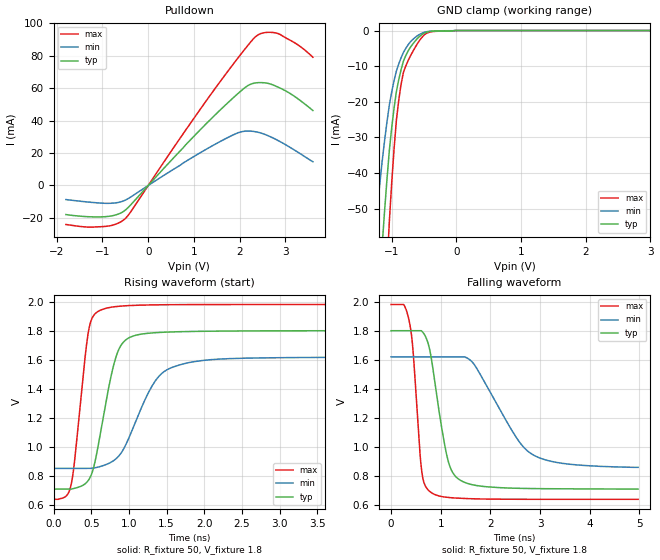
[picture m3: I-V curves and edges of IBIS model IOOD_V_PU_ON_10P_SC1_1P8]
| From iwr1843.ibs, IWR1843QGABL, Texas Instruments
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|   Model Cell IOOD_V_PU_ON_10P_SC1_1P8
|IOOD_V_PU_ON_10P_SC1_1P8
[Model]   IOOD_V_PU_ON_10P_SC1_1P8
Model_type   I/O_open_drain
Polarity   Non-Inverting
Enable   Active-Low
Vinl =  0.63
Vinh =  1.17
Cref =  15pF
Rref =  100.0000M
Vref =  0V
Vmeas =  0.9
|   typ   min   max
C_comp   2.290246p   2.205796p   2.292736p
[Model Spec]
Vinl   0.63   0.567   0.693
Vinh   1.17   1.053   1.287
[Temperature Range]   25   125   -40
[Voltage Range]   1.8   1.62   1.98
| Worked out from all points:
|   slope of the pulldown table from 0 to 0.27 V, typ, clamps not added: 32.2 ohm
|   GND clamp passes 1 mA (typ) near -0.52 V on its own axis
|   rising waveform, R_fixture 50, V_fixture 1.8: 20-80 % time 245ps typ, 416ps min, 160ps max; typ from 0.711 V to 1.8 V
|   falling waveform, R_fixture 50, V_fixture 1.8: 20-80 % time 308ps typ, 788ps min, 165ps max; typ from 1.8 V to 0.71 V
| Where Nom  PVT is Nominal Process, 1.8V, 25C
|   Fast PVT is Strong Process,  1.98V, -40C
|   Slow PVT is Weak Process,   1.62V, 125C
[Pulldown]
|   voltage   I(typ)   I(min)   I(max)
-1.8V     -17.92mA   -8.674mA   -24.03mA
-927.3mV  -19.22mA   -10.99mA   -25.21mA
-654.5mV  -17.65mA   -10.46mA   -23.22mA
-490.9mV  -14.97mA   -8.904mA   -20.12mA
818.2mV   25.06mA    14.78mA    34.16mA
1.691V    49.7mA     28.87mA    68.59mA
2.127V    60.63mA    33.53mA    84.59mA
2.4V      63.43mA    32.84mA    92.9mA
2.618V    62.99mA    30.74mA    94.47mA
2.836V    60.69mA    27.76mA    93.76mA
3.273V    53.49mA    20.53mA    86.73mA
3.6V      46.26mA    14.64mA    79.12mA
[GND_clamp]
|   voltage   I(typ)   I(min)   I(max)
-1.8V     -270.2mA   -170.2mA   -430.1mA
-1.255V   -91.68mA   -55.92mA   -148.5mA
-1.145V   -59.94mA   -36.46mA   -97.15mA
-1.109V   -50.51mA   -30.84mA   -81.62mA
-1.073V   -41.77mA   -25.67mA   -67.14mA
-1.036V   -33.71mA   -20.94mA   -53.69mA
-927.3mV  -17.15mA   -11.38mA   -25.2mA
-854.5mV  -10.96mA   -7.657mA   -15.09mA
-781.8mV  -7.031mA   -4.995mA   -9.958mA
-563.6mV  -1.569mA   -1.036mA   -2.651mA
-18.18mV  0A         0A         0A
3.6V      0A         0A         0A
[Ramp]
| variable   typ   min   max
dV/dt_f 0.66095897/0.31060812n 0.46741276/0.81020272n 0.80998719/0.16631685n
dV/dt_r 0.65862638/0.43190449n 0.47366209/1.0494131n 0.81474121/0.23003732n
R_load = 50
[Rising Waveform]
R_fixture = 50
V_fixture = 1.8
V_fixture_min = 1.62
V_fixture_max = 1.98
|   time   V(typ)   V(min)   V(max)
0s        710.6mV    852.8mV    640.5mV
228.8ps   710.6mV    852.8mV    730.4mV
277.8ps   716.3mV    852.8mV    897.5mV
460.2ps   769.7mV    852.8mV    1.785V
608.1ps   1.054V     864.3mV    1.937V
831.2ps   1.624V     920.4mV    1.966V
1.058ns   1.764V     1.135V     1.974V
1.377ns   1.787V     1.474V     1.978V
1.755ns   1.794V     1.576V     1.979V
4.974ns   1.8V       1.618V     1.98V
[Falling Waveform]
R_fixture = 50
V_fixture = 1.8
V_fixture_min = 1.62
V_fixture_max = 1.98
|   time   V(typ)   V(min)   V(max)
0s        1.8V       1.62V      1.981V
368.4ps   1.8V       1.62V      1.86V
440.1ps   1.8V       1.62V      1.67V
613.3ps   1.799V     1.62V      843.1mV
788ps     1.653V     1.62V      690.9mV
1.123ns   939.8mV    1.62V      653.8mV
1.375ns   775.1mV    1.62V      647mV
1.663ns   738.3mV    1.573V     643.3mV
2.826ns   713.9mV    953mV      639.9mV
4.974ns   710.1mV    859.9mV    639.7mV
